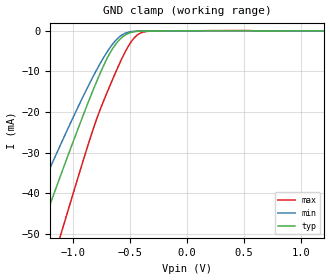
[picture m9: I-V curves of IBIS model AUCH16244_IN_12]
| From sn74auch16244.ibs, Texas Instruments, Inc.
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[Model]   AUCH16244_IN_12
Model_type  Input
Vinl=0.385
Vinh=0.845
| variable   typ   min   max
C_comp   3.46pF   2.83pF   4.05pF
[Temperature Range]   40   100   -40
| Ambient temperature   25   85   -40
[Voltage range]   1.2   1.1   1.3
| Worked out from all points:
|   GND clamp passes 1 mA (typ) near -0.54 V on its own axis
[GND Clamp]
| AUCH16244_IN_12
|   Voltage   I(typ)   I(min)   I(max)
-3.6V     -232.7mA   -194.4mA   -280.6mA
-1.46V    -62.8mA    -50.19mA   -83.06mA
-1.415V   -59.27mA   -47.29mA   -78.85mA
-1.285V   -49.13mA   -38.97mA   -66.69mA
-1.12V    -36.41mA   -28.64mA   -51.26mA
-1.085V   -33.74mA   -26.49mA   -48mA
-830mV    -15mA      -11.57mA   -24.72mA
-685mV    -5.916mA   -4.511mA   -14.07mA
-570mV    -1.619mA   -1.012mA   -6.745mA
-440mV    -150.9uA   -79.3uA    -1.112mA
-300mV    -34.37uA   -20.85uA   -74.27uA
1.2V      152.4pA    533.5nA    33.85pA
